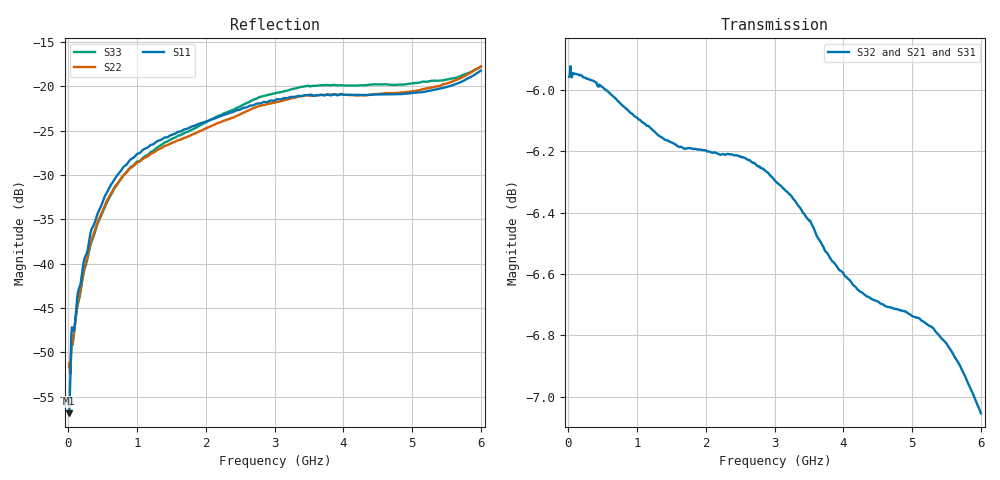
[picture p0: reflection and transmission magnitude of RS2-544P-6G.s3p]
! MTS Systemtechnik GmbH
! S-Parameters
! Model: RS2-544P-6G
! Rohde & Schwarz ZVB8 2Ports - Version 3.20 - 1145.1010k08 SN: 100119
! Converted & adapted with MATLAB
!		|  MTS  |
!		|  |--o OUT 2 (Port 3)
! C (Port 1) o--| RS2-544P-6G |
!		|  |--o OUT 1 (Port 2)
! S3P File: Measurements:
! <S11,S12,S13>,
! <S21,S22,S23>,
! <S31,S32,S33>:
# HZ  S  DB  R  50.00
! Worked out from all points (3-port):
!   600 points, 10 MHz to 6 GHz, reference 50 ohm
!   strongest paths, dB at 10 MHz, 1.51 GHz, 3.01 GHz, 4.51 GHz, 6 GHz:
!     S32: -6.0, -6.2, -6.3, -6.7, -7.1
!     S21: -6.0, -6.2, -6.3, -6.8, -7.2
!     S31: -6.0, -6.2, -6.3, -6.8, -7.2
!   lowest |S11| = -56.9 dB at 10 MHz (marker M1), VSWR 1.00, Z = 50.1 - j0.0485 ohm
!   |S11| at or under -10 dB: start of sweep to end of sweep
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1e7  -56.87 -19.7  -5.98 -0.8  -5.99 -0.8
     -5.97 -0.8  -51.22 -11.4  -5.98 -0.8
     -5.97 -0.8  -5.96 -0.7  -51.51 -11.6
7e7  -47.56 -38.4  -5.98 -6.2  -5.98 -6.2
     -5.97 -6.1  -48.38 -41.5  -5.98 -6.2
     -5.96 -6.1  -5.94 -6.1  -48.58 -41.6
2.3e8  -39.52 -87.0  -6.00 -20.3  -6.00 -20.4
       -5.98 -20.3  -40.55 -87.1  -5.99 -20.4
       -5.98 -20.3  -5.96 -20.3  -40.72 -88.6
7e8  -30.13 -139.3  -6.06 -61.8  -6.07 -61.9
     -6.05 -61.7  -31.10 -142.7  -6.06 -61.9
     -6.05 -61.9  -6.03 -61.8  -31.18 -146.9
1.27e9  -26.31 172.2  -6.16 -111.6  -6.18 -111.7
        -6.15 -111.5  -27.30 166.2  -6.18 -111.8
        -6.15 -111.7  -6.14 -111.7  -27.03 159.6
1.95e9  -24.13 117.5  -6.21 -170.9  -6.23 -171.1
        -6.20 -170.9  -24.93 111.1  -6.23 -171.0
        -6.21 -171.0  -6.20 -170.9  -24.27 104.5
3.01e9  -21.57 23.6  -6.35 95.1  -6.37 94.9
        -6.34 95.1  -21.82 24.5  -6.33 95.3
        -6.34 95.0  -6.30 95.4  -20.78 23.0
4.2e9  -20.99 -76.6  -6.75 -10.0  -6.77 -10.2
       -6.75 -10.0  -21.05 -69.5  -6.65 -9.5
       -6.77 -10.2  -6.65 -9.5  -19.93 -68.8
5.1e9  -20.68 -125.2  -6.86 -90.2  -6.90 -90.5
       -6.86 -90.2  -20.45 -117.4  -6.74 -89.8
       -6.90 -90.5  -6.74 -89.8  -19.60 -120.6
6e9  -18.23 -154.2  -7.17 -173.3  -7.24 -173.4
     -7.17 -173.3  -17.74 -148.1  -7.05 -172.5
     -7.24 -173.4  -7.05 -172.6  -17.81 -153.9
